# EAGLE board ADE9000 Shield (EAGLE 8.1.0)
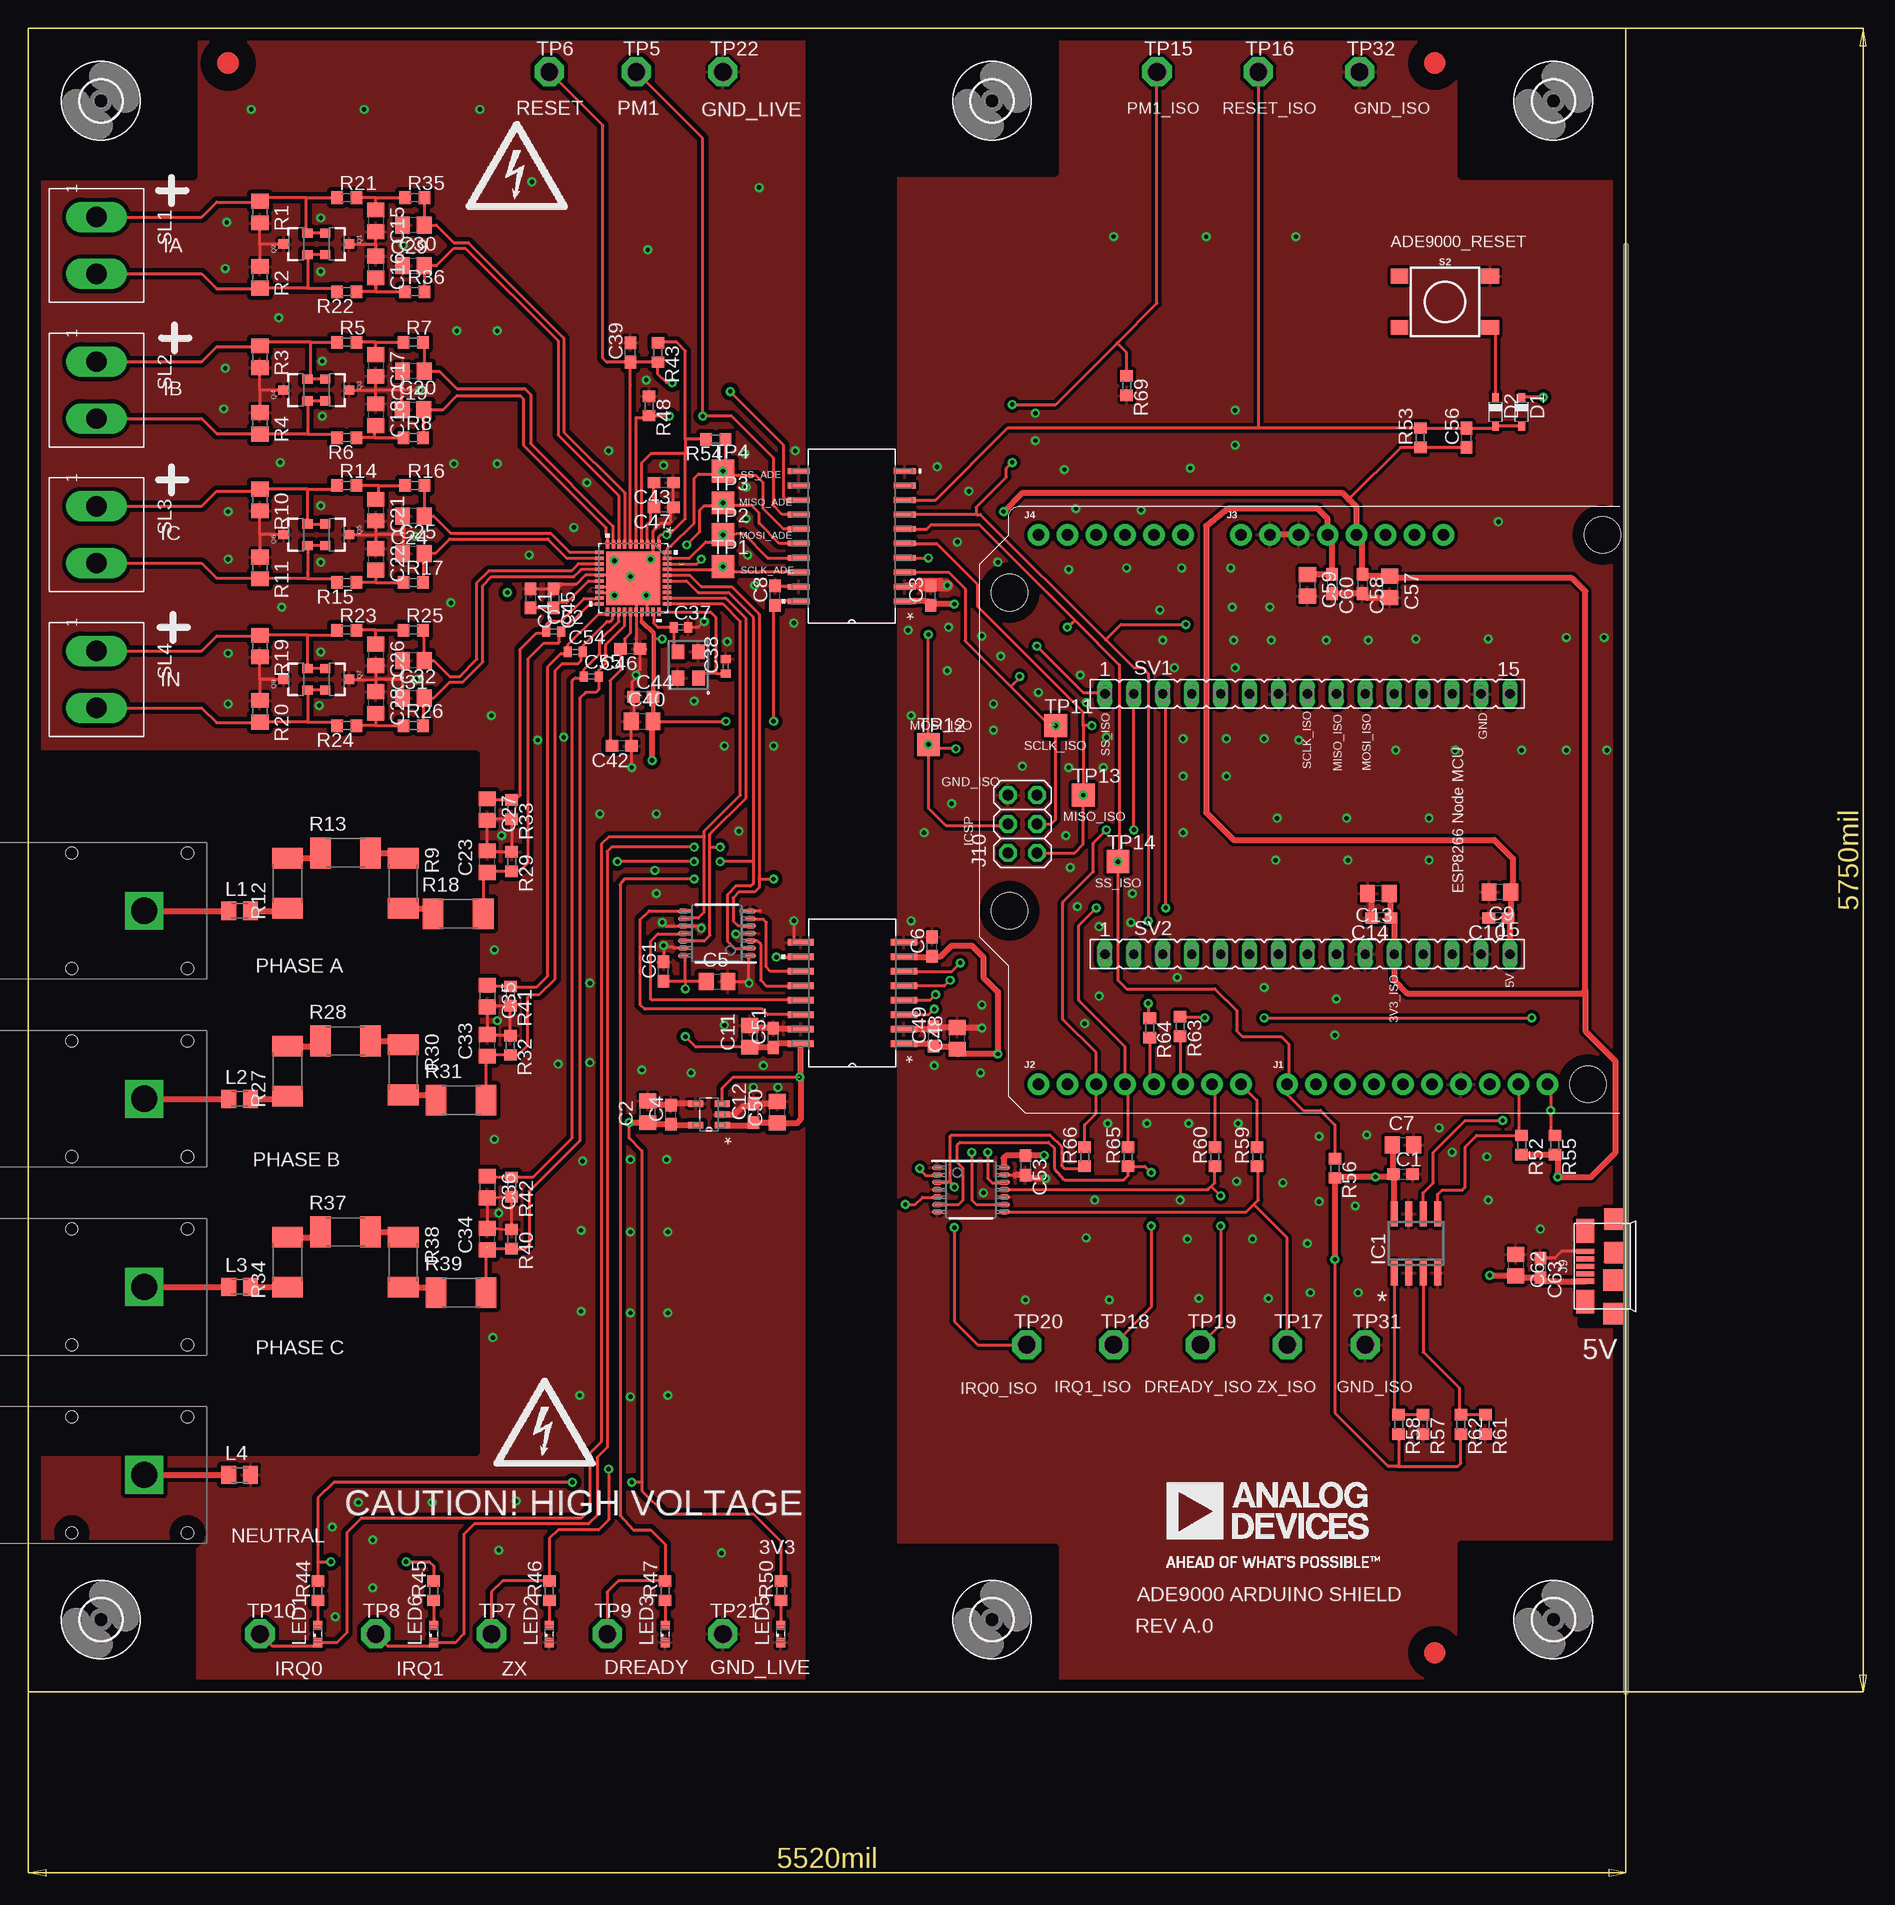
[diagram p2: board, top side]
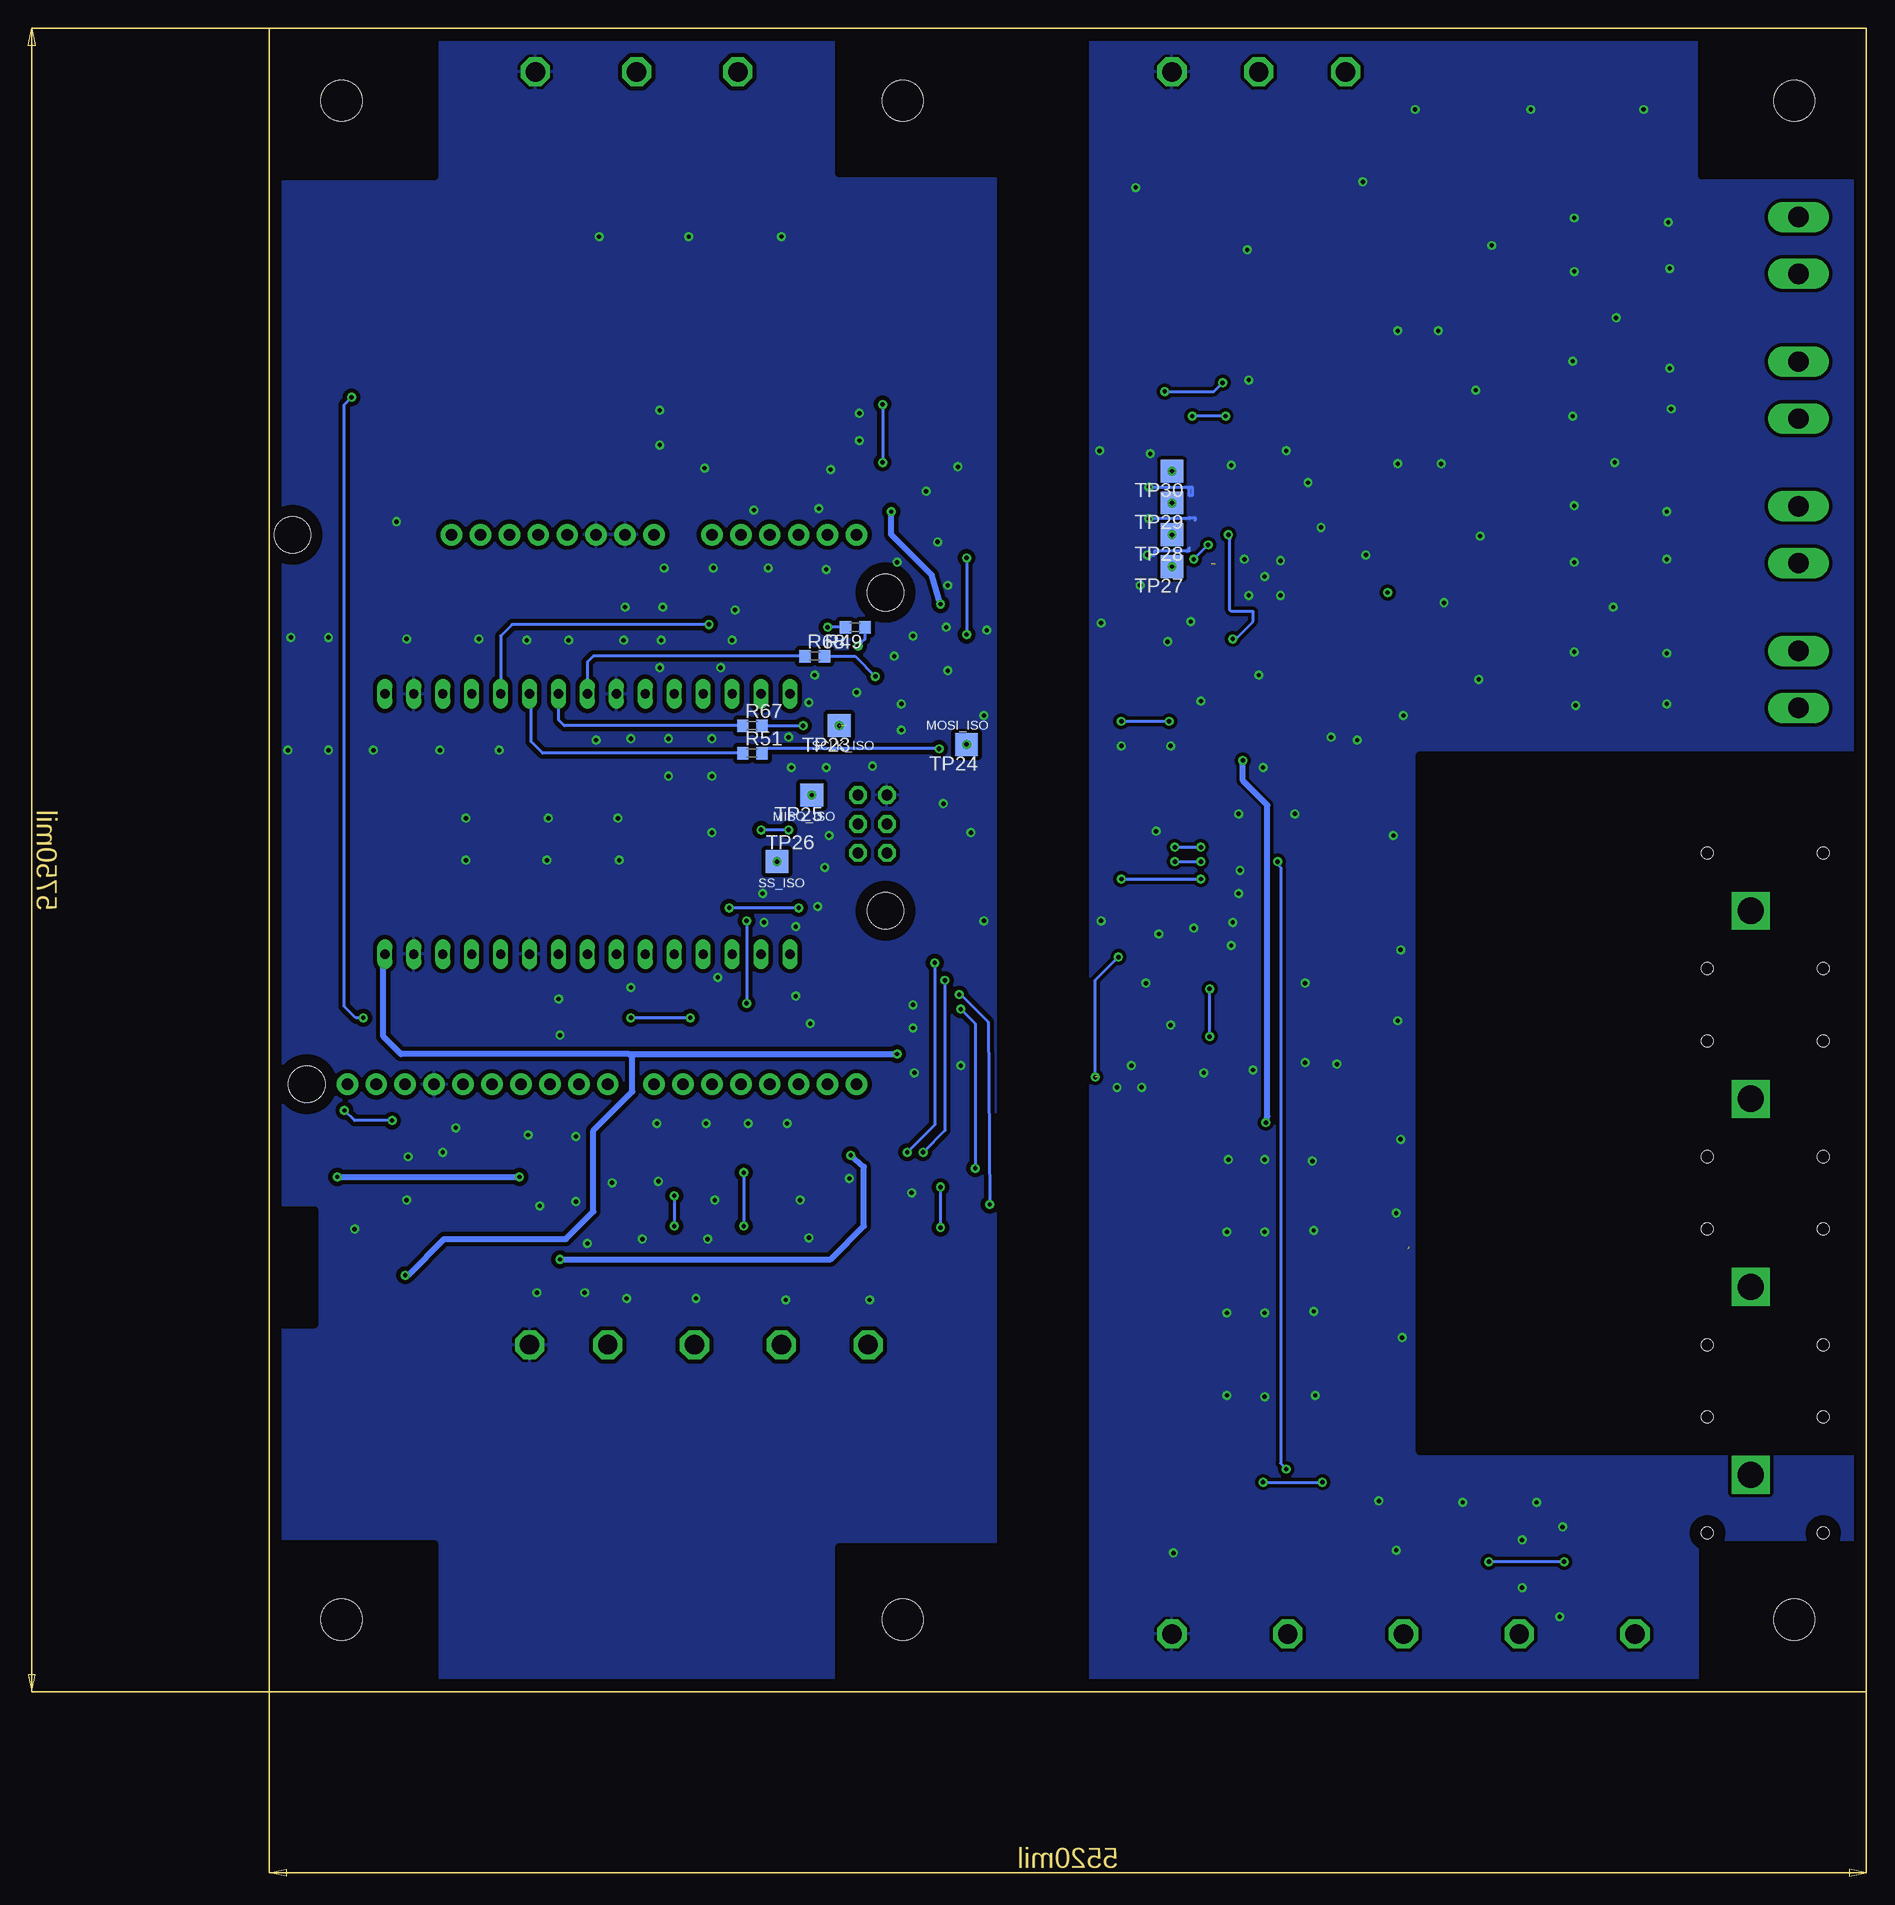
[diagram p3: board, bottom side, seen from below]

Size 161.34 x 162.23 mm. Coordinates in mm from the lower left corner, seen from the top.
Outline: 0,16.18 140.21,16.18 140.21,162.23 0,162.23 0,16.18
Copper layers (1*16): Top 0.035mm / dielectric 1.5mm / Bottom 0.035mm
Design rules "default": minimum track width 10mil, minimum drill 24mil, track to track 8mil, track to pad 8mil, pad to pad 8mil, via to via 8mil, smd to smd 8mil, copper to edge 40mil, drill to drill 8mil, minimum pad ring 10mil, minimum via ring 8mil, stop-mask expansion 4mil, vias tented up to drill 0mil, thermal gap 10mil
Holes 3.2 mm at 136.91,69.52 86.11,84.75 86.11,112.69 138.18,117.77
tRestrict: area 0,37.3 to 39.2,98.5; area 68.6,111.7 to 75.9,125.9; area 68.6,82.3 to 75.9,82.5; area 69,72.6 to 75.7,82.3; area 68.6,16.2 to 75.9,72.6; area 68.6,82.3 to 75.9,162.2; area 0.1,16.4 to 14.4,29.1; area 125.7,16.4 to 140,29.1; area 125.7,149.3 to 140,162; area 0.3,149.3 to 14.5,162; area 136.3,48.4 to 139.3,58.5; area 75.9,16.2 to 90.2,28.9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
bRestrict: area 0,37.3 to 39.2,98.5; area 68.6,16.2 to 75.9,162.2; area 0.1,16.4 to 14.4,29.1; area 125.7,16.4 to 140,29.1; area 125.7,149.3 to 140,162; area 0.3,149.3 to 14.5,162; area 136.3,48.4 to 139.3,58.5; area 75.9,16.2 to 90.2,28.9; area 75.9,149.5 to 90.2,162.2

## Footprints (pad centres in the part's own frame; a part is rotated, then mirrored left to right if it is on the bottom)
C0603 = smd 1.1 x 1: 1 -0.85,0; 2 0.85,0
C0805 = smd 1.3 x 1.5: 1 -0.95,0; 2 0.95,0
C0402 = smd 0.7 x 0.9: 1 -0.65,0; 2 0.65,0
SOD323_ST = smd 0.8 x 0.6: A 1.25,0; C -1.25,0
3,6 = hole 3.6: 0,0
SO-08 = smd 0.6 x 2.2: 1 -1.905,-2.6; 2 -0.635,-2.6; 3 0.635,-2.6; 4 1.905,-2.6; 5 1.905,2.6; 6 0.635,2.6; 7 -0.635,2.6; 8 -1.905,2.6
1X10_NO_SILK = drill 1.016 pad 1.88: 1 0,0; 2 2.54,0; 3 5.08,0; 4 7.62,0; 5 10.16,0; 6 12.7,0; 7 15.24,0; 8 17.78,0; 9 20.32,0; 10 22.86,0
1X08_NO_SILK = drill 1.016 pad 1.88: 1 0,0; 2 2.54,0; 3 5.08,0; 4 7.62,0; 5 10.16,0; 6 12.7,0; 7 15.24,0; 8 17.78,0
1X06_NO_SILK = drill 1.016 pad 1.88: 1 0,0; 2 2.54,0; 3 5.08,0; 4 7.62,0; 5 10.16,0; 6 12.7,0
SLB4-I/90 = drill 2.305 pad 2.794 square: P$1 0,0 | hole 1.054: -3.8,-5.08; -3.8,5.08; 6.36,5.08; 6.36,-5.08
USB-MICRO-10103594 = smd 0.4 x 1.6: D+ 0,0; D- -0.65,0; GND 1.3,0; ID 0.65,0; VBUS -1.3,0 | smd 1.9 x 1.9: SHLD1 -1.2,-2.55; SHLD2 1.2,-2.55; SHLD3 -4.15,-2.55; SHLD4 4.15,-2.55 | smd 2.1 x 1.6: SHLD5 3.1,0; SHLD6 -3.1,0
ARDUINO_2X03 = drill 0.95 pad 1.55 octagon: 1 -2.54,-1.27; 2 -2.54,1.27; 3 0,-1.27; 4 0,1.27; 5 2.54,-1.27; 6 2.54,1.27
M0805 = smd 1.3 x 1.6: 1 -0.95,0; 2 0.95,0
SML0603 = smd 0.8 x 0.8: A 0.75,0; C -0.75,0
SOT23-3 = smd 0.8 x 0.9: 1 -0.95,-1; 2 0.95,-1; 3 0,1.1
SMD_4PIN_3.2X2.1 = smd 1.3 x 1.1: 1 -1.15,-0.9; 2 1.15,-0.9; 3 1.15,0.9; 4 -1.15,0.9
R0805 = smd 1.3 x 1.5: 1 -0.95,0; 2 0.95,0
R0603 = smd 1 x 1.1: 1 -0.85,0; 2 0.85,0
R2010 = smd 1.8 x 2.7: 1 -2.2,0; 2 2.2,0
TACTILE_SWITCH_SMD_6.2MM_TALL = smd 1.55 x 1.3: A1 -3.975,-2.25; A2 3.975,-2.25; B1 -3.975,2.25; B2 3.975,2.25
02P = drill 1.778 long: 1 -2.5,0; 2 2.5,0
FE15 = drill 0.813 long: 1 -17.78,0; 2 -15.24,0; 3 -12.7,0; 4 -10.16,0; 5 -7.62,0; 6 -5.08,0; 7 -2.54,0; 8 0,0; 9 2.54,0; 10 5.08,0; 11 7.62,0; 12 10.16,0; 13 12.7,0; 14 15.24,0; 15 17.78,0
TP20SQ = smd 2 x 2: TP 0,0
P1-17 = drill 1.702 pad 2.54 octagon: TP 0,0
CP_40_7 = smd 0.762 x 0.305: 1 -2.972,2.25; 2 -2.972,1.75; 3 -2.972,1.25; 4 -2.972,0.75; 5 -2.972,0.25; 6 -2.972,-0.25; 7 -2.972,-0.75; 8 -2.972,-1.25; 9 -2.972,-1.75; 10 -2.972,-2.25; 21 2.972,-2.25; 22 2.972,-1.75; 23 2.972,-1.25; 24 2.972,-0.75; 25 2.972,-0.25; 26 2.972,0.25; 27 2.972,0.75; 28 2.972,1.25; 29 2.972,1.75; 30 2.972,2.25 | smd 0.305 x 0.762: 11 -2.25,-2.972; 12 -1.75,-2.972; 13 -1.25,-2.972; 14 -0.75,-2.972; 15 -0.25,-2.972; 16 0.25,-2.972; 17 0.75,-2.972; 18 1.25,-2.972; 19 1.75,-2.972; 20 2.25,-2.972; 31 2.25,2.972; 32 1.75,2.972; 33 1.25,2.972; 34 0.75,2.972; 35 0.25,2.972; 36 -0.25,2.972; 37 -0.75,2.972; 38 -1.25,2.972; 39 -1.75,2.972; 40 -2.25,2.972 | smd 4.699 x 4.699: 41 0,0
RI_16_1 = smd 2.306 x 0.561: 1 -4.527,4.445; 2 -4.527,3.175; 3 -4.527,1.905; 4 -4.527,0.635; 5 -4.527,-0.635; 6 -4.527,-1.905; 7 -4.527,-3.175; 8 -4.527,-4.445; 9 4.527,-4.445; 10 4.527,-3.175; 11 4.527,-1.905; 12 4.527,-0.635; 13 4.527,0.635; 14 4.527,1.905; 15 4.527,3.175; 16 4.527,4.445
PW0014A_N = smd 0.95 x 0.45: 1 -2.95,1.95; 2 -2.95,1.3; 3 -2.95,0.65; 4 -2.95,0; 5 -2.95,-0.65; 6 -2.95,-1.3; 7 -2.95,-1.95; 8 2.95,-1.95; 9 2.95,-1.3; 10 2.95,-0.65; 11 2.95,0; 12 2.95,0.65; 13 2.95,1.3; 14 2.95,1.95
UJ_5 = smd 1.321 x 0.559: 1 -1.168,0.95; 2 -1.168,0; 3 -1.168,-0.95; 4 1.168,-0.95; 5 1.168,0.95
RI_20_1 = smd 1.921 x 0.511: 1 -4.65,5.715; 2 -4.65,4.445; 3 -4.65,3.175; 4 -4.65,1.905; 5 -4.65,0.635; 6 -4.65,-0.635; 7 -4.65,-1.905; 8 -4.65,-3.175; 9 -4.65,-4.445; 10 -4.65,-5.715; 11 4.65,-5.715; 12 4.65,-4.445; 13 4.65,-3.175; 14 4.65,-1.905; 15 4.65,-0.635; 16 4.65,0.635; 17 4.65,1.905; 18 4.65,3.175; 19 4.65,4.445; 20 4.65,5.715

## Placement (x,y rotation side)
C1  0.1u  [C0603]  120.65,61.64 0 top
C2  10u  [C0805]  54.36,67.1 90 top
C3  0.1u  [C0603]  79.2,112.44 90 top
C4  0.1u  [C0603]  56.39,66.85 90 top
C5  4.7u  [C0805]  60.45,78.53 0 top
C6  0.1u  [C0603]  79.32,81.61 90 top
C7  4.7u  [C0805]  120.65,64.18 0 top
C8  0.1u  [C0603]  65.53,112.44 90 top
C9  10u  [C0805]  129.16,86.41 180 top
C10  0.1u  [C0603]  129.03,84.12 180 top
C11  10u  [C0805]  63.3,73.73 90 top
C12  0.1u  [C0603]  63.65,67 90 top
C13  10u  [C0805]  118.49,86.28 180 top
C14  0.1u  [C0603]  118.75,84.12 180 top
C15  DNP  [C0805]  30.48,145.33 270 top
C16  DNP  [C0805]  30.48,141.27 270 top
C17  DNP  [C0805]  30.48,132.63 270 top
C18  DNP  [C0805]  30.48,128.32 270 top
C19  0.022u  [C0805]  33.78,132.13 180 top
C20  0.022u  [C0805]  33.76,128.77 0 top
C21  DNP  [C0805]  30.48,119.93 270 top
C22  DNP  [C0805]  30.48,115.62 270 top
C23  0.022u  [C0805]  40.26,89.07 90 top
C24  0.022u  [C0805]  33.78,119.43 180 top
C25  0.022u  [C0805]  33.78,116.12 0 top
C26  DNP  [C0805]  30.48,107.23 270 top
C27  0.022u  [C0805]  40.26,93.64 270 top
C28  DNP  [C0805]  30.48,103.04 270 top
C29  0.022u  [C0805]  33.78,144.95 180 top
C30  0.022u  [C0805]  33.78,141.4 0 top
C31  0.022u  [C0805]  33.78,106.73 180 top
C32  0.022u  [C0805]  33.78,103.42 0 top
C33  0.022u  [C0805]  40.26,72.94 90 top
C34  0.022u  [C0805]  40.26,55.93 90 top
C35  0.022u  [C0805]  40.26,77.26 270 top
C36  0.022u  [C0805]  40.26,60.5 270 top
C37  18p  [C0402]  57.28,109.65 0 top
C38  18p  [C0402]  61.21,106.22 90 top
C39  1u  [C0603]  52.83,133.78 90 top
C40  4.7u  [C0805]  53.87,101.39 0 top
C41  4.7u  [C0603]  44.07,112.19 270 top
C42  4.7u  [C0603]  52.07,99.23 180 top
C43  4.7u  [C0603]  55.75,122.35 180 top
C44  0.1u  [C0603]  53.98,103.55 0 top
C45  0.1u  [C0603]  46.1,112.19 270 top
C46  0.1u  [C0603]  52.83,107.74 180 top
C47  0.1u  [C0603]  55.75,120.19 180 top
C48  10u  [C0805]  81.53,73.55 90 top
C49  0.1u  [C0603]  79.45,73.71 90 top
C50  10u  [C0805]  65.74,67.08 90 top
C51  0.1u  [C0603]  65.38,73.6 90 top
C52  51p  [C0402]  46.1,109.27 0 top
C53  0.1u  [C0603]  87.5,62.4 270 top
C54  51p  [C0402]  48.01,107.49 0 top
C55  51p  [C0402]  49.4,105.33 0 top
C56  1u  [C0603]  126.24,126.28 90 top
C57  10u  [C0805]  119.51,113.2 270 top
C58  0.1u  [C0603]  117.09,113.46 270 top
C59  10u  [C0805]  112.27,113.33 270 top
C60  0.1u  [C0603]  114.43,113.46 270 top
C61  0.1u  [C0603]  55.75,79.42 90 top
C62  22u  [C0805]  130.56,53.64 270 top
C63  0.1u  [C0603]  132.72,53.39 270 top
D1  BAT54WS  [SOD323_ST]  131.06,128.57 270 top
D2  BAT54WS  [SOD323_ST]  128.78,128.57 270 top
DRILEGEND  [DRILEGEND]  not placed on the board
H1  MOUNT-HOLE3.6  [3,6]  6.35,22.52 0 top
H2  MOUNT-HOLE3.6  [3,6]  6.35,155.88 0 top
H3  MOUNT-HOLE3.6  [3,6]  133.86,155.88 0 top
H4  MOUNT-HOLE3.6  [3,6]  133.86,22.52 0 top
H5  MOUNT-HOLE3.6  [3,6]  84.58,22.52 0 top
H6  MOUNT-HOLE3.6  [3,6]  84.58,155.88 0 top
IC1  24LC32A/SN  [SO-08]  121.79,55.55 0 top
J1  [1X10_NO_SILK]  110.49,69.52 0 top
J2  [1X08_NO_SILK]  88.65,69.52 0 top
J3  [1X08_NO_SILK]  106.43,117.77 0 top
J4  [1X06_NO_SILK]  88.65,117.77 0 top
J5  23.3200-22  [SLB4-I/90]  10.16,84.75 180 top
J6  23.3200-22  [SLB4-I/90]  10.16,68.25 180 top
J7  23.3200-22  [SLB4-I/90]  10.16,51.73 180 top
J8  23.3200-21  [SLB4-I/90]  10.16,35.23 180 top
J9  ZX62-AB-5PA(31)  [USB-MICRO-10103594]  136.65,53.54 90 top
J10  [ARDUINO_2X03]  87.25,92.38 90 top
L1  1500  [M0805]  18.54,84.75 0 top
L2  1500  [M0805]  18.54,68.25 0 top
L3  1500  [M0805]  18.54,51.73 0 top
L4  1500  [M0805]  18.54,35.23 0 top
LED1  APT1608LSECK/J3-PRV  [SML0603]  25.4,21.26 90 top
LED2  APT1608LSECK/J3-PRV  [SML0603]  45.72,21.26 90 top
LED3  APT1608LSECK/J3-PRV  [SML0603]  55.88,21.26 90 top
LED5  APT1608LZGCK  [SML0603]  66.04,21.26 90 top
LED6  APT1608LSECK/J3-PRV  [SML0603]  35.56,21.26 90 top
Q1  MMBD4148SE  [SOT23-3]  27.05,143.3 270 top
Q2  MMBD4148SE  [SOT23-3]  23.5,143.3 90 top
Q3  MMBD4148SE  [SOT23-3]  27.05,130.47 270 top
Q4  MMBD4148SE  [SOT23-3]  23.5,130.47 90 top
Q5  MMBD4148SE  [SOT23-3]  27.05,117.77 270 top
Q6  MMBD4148SE  [SOT23-3]  23.5,117.77 90 top
Q7  MMBD4148SE  [SOT23-3]  27.05,105.08 270 top
Q8  ECS-245.7-12-33Q-JES-TR  [SMD_4PIN_3.2X2.1]  57.91,106.34 90 top
Q9  MMBD4148SE  [SOT23-3]  23.5,105.08 90 top
R1  5.1  [R0805]  20.32,146.1 270 top
R2  5.1  [R0805]  20.32,140.38 270 top
R3  5.1  [R0805]  20.32,133.4 270 top
R4  5.1  [R0805]  20.32,127.55 270 top
R5  0  [R0603]  27.94,134.67 0 top
R6  0  [R0603]  27.94,126.28 180 top
R7  1k  [R0603]  33.78,134.67 0 top
R8  1k  [R0603]  33.78,126.28 0 top
R9  200k  [R2010]  32.89,87.17 270 top
R10  5.1  [R0805]  20.32,120.82 270 top
R11  5.1  [R0805]  20.32,114.85 270 top
R12  200k  [R2010]  22.73,87.17 90 top
R13  200k  [R2010]  27.81,89.83 0 top
R14  0  [R0603]  27.94,122.09 0 top
R15  0  [R0603]  27.94,113.58 180 top
R16  1k  [R0603]  33.91,122.09 0 top
R17  1k  [R0603]  33.78,113.58 0 top
R18  200k  [R2010]  37.72,84.5 0 top
R19  5.1  [R0805]  20.32,108 270 top
R20  5.1  [R0805]  20.32,102.28 270 top
R21  0  [R0603]  27.94,147.37 0 top
R22  0  [R0603]  27.94,139.11 180 top
R23  0  [R0603]  27.94,109.39 0 top
R24  0  [R0603]  27.94,101.01 180 top
R25  1k  [R0603]  33.78,109.39 0 top
R26  1k  [R0603]  33.78,101.01 0 top
R27  200k  [R2010]  22.73,70.66 90 top
R28  200k  [R2010]  27.81,73.33 0 top
R29  1k  [R0603]  42.42,89.07 270 top
R30  200k  [R2010]  32.89,70.78 270 top
R31  200k  [R2010]  37.97,68.12 0 top
R32  1k  [R0603]  42.29,72.94 270 top
R33  1k  [R0603]  42.42,93.64 270 top
R34  200k  [R2010]  22.73,53.89 90 top
R35  1k  [R0603]  33.91,147.37 0 top
R36  1k  [R0603]  33.91,139.11 0 top
R37  200k  [R2010]  27.81,56.56 0 top
R38  200k  [R2010]  32.89,53.89 270 top
R39  200k  [R2010]  37.97,51.23 0 top
R40  1k  [R0603]  42.42,55.93 270 top
R41  1k  [R0603]  42.29,77.26 270 top
R42  1k  [R0603]  42.42,60.5 270 top
R43  10k  [R0603]  55.24,133.78 270 top
R44  3k  [R0603]  25.4,25.07 90 top
R45  3k  [R0603]  35.56,25.07 90 top
R46  3k  [R0603]  45.72,25.07 90 top
R47  3k  [R0603]  55.88,25.07 90 top
R48  10k  [R0603]  54.48,129.08 270 top
R49  DNP  [R0603]  88.77,109.65 180 bottom
R50  3k  [R0603]  66.04,25.07 90 top
R51  DNP  [R0603]  97.79,98.6 0 bottom
R52  10k  [R0603]  131.06,64.18 270 top
R53  10k  [R0603]  122.17,126.28 90 top
R54  10k  [R0603]  60.33,126.16 180 top
R55  10k  [R0603]  133.99,64.18 270 top
R56  10k  [R0603]  114.68,62.15 270 top
R57  0  [R0603]  122.43,39.67 270 top
R58  DNP  [R0603]  120.27,39.67 270 top
R59  0  [R0603]  107.82,63.17 90 top
R60  0  [R0603]  104.14,63.17 90 top
R61  DNP  [R0603]  127.89,39.67 270 top
R62  0  [R0603]  125.73,39.67 270 top
R63  0  [R0603]  101.09,74.59 270 top
R64  0  [R0603]  98.42,74.47 270 top
R65  0  [R0603]  96.52,63.17 90 top
R66  0  [R0603]  92.71,63.17 90 top
R67  DNP  [R0603]  97.79,101.01 0 bottom
R68  DNP  [R0603]  92.33,107.11 0 bottom
R69  10k  [R0603]  96.39,130.86 270 top
S2  PTS645SM43SMTR92  [TACTILE_SWITCH_SMD_6.2MM_TALL]  124.33,138.22 0 top
SL1  25.161.0253.0  [02P]  5.97,143.18 270 top
SL2  25.161.0253.0  [02P]  5.97,130.47 270 top
SL3  25.161.0253.0  [02P]  5.97,117.77 270 top
SL4  25.161.0253.0  [02P]  5.97,105.08 270 top
SV1  DNI  [FE15]  112.27,103.8 0 top
SV2  DNI  [FE15]  112.27,80.94 0 top
TP1  TPTP20SQ  [TP20SQ]  60.96,114.98 0 top
TP2  TPTP20SQ  [TP20SQ]  60.96,117.77 0 top
TP3  TPTP20SQ  [TP20SQ]  60.96,120.57 0 top
TP4  TPTP20SQ  [TP20SQ]  60.96,123.36 0 top
TP5  TPPAD1-17  [P1-17]  53.34,158.42 0 top
TP6  TPPAD1-17  [P1-17]  45.72,158.42 0 top
TP7  TPPAD1-17  [P1-17]  40.64,21.26 0 top
TP8  TPPAD1-17  [P1-17]  30.48,21.26 0 top
TP9  TPPAD1-17  [P1-17]  50.8,21.26 0 top
TP10  TPPAD1-17  [P1-17]  20.32,21.26 0 top
TP11  TPTP20SQ  [TP20SQ]  90.17,101.01 0 top
TP12  TPTP20SQ  [TP20SQ]  78.99,99.36 0 top
TP13  TPTP20SQ  [TP20SQ]  92.58,94.91 0 top
TP14  TPTP20SQ  [TP20SQ]  95.63,89.07 0 top
TP15  TPPAD1-17  [P1-17]  99.06,158.42 0 top
TP16  TPPAD1-17  [P1-17]  107.95,158.42 0 top
TP17  TPPAD1-17  [P1-17]  110.49,46.66 0 top
TP18  TPPAD1-17  [P1-17]  95.25,46.66 0 top
TP19  TPPAD1-17  [P1-17]  102.87,46.66 0 top
TP20  TPPAD1-17  [P1-17]  87.63,46.66 0 top
TP21  TPPAD1-17  [P1-17]  60.96,21.26 0 top
TP22  TPPAD1-17  [P1-17]  60.96,158.42 0 top
TP23  TPTP20SQ  [TP20SQ]  90.17,101.01 180 bottom
TP24  TPTP20SQ  [TP20SQ]  78.99,99.36 180 bottom
TP25  TPTP20SQ  [TP20SQ]  92.58,94.91 180 bottom
TP26  TPTP20SQ  [TP20SQ]  95.63,89.07 0 bottom
TP27  TPTP20SQ  [TP20SQ]  60.96,114.98 180 bottom
TP28  TPTP20SQ  [TP20SQ]  60.96,117.77 180 bottom
TP29  TPTP20SQ  [TP20SQ]  60.96,120.57 180 bottom
TP30  TPTP20SQ  [TP20SQ]  60.96,123.36 180 bottom
TP31  TPPAD1-17  [P1-17]  117.35,46.66 0 top
TP32  TPPAD1-17  [P1-17]  116.84,158.42 0 top
U1  ADE9000ACPZ  [CP_40_7]  53.09,113.97 270 top
U2  ADUM6404ARIZ  [RI_16_1]  72.31,77.54 180 top
U3  SN74LV4T125PWR  [PW0014A_N]  60.43,82.77 180 top
U4  ADP122AUJZ-3.3-R7  [UJ_5]  59.74,66.87 180 top
U5  ADUM4151BRIZ  [RI_20_1]  72.26,117.65 180 top
U6  SN74LV4T125PWR  [PW0014A_N]  82.73,60.27 0 top

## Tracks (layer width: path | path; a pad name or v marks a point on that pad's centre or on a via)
5V_ADE  (via drill 0.38)  (1 unrouted)
  Top 0.254: U4.3 60.91,69.21 61.85,70.15 67.53,70.15 67.79,70.4 | v65.66,80.69 67.76,80.69 U2.10 | C11.1 58.58,72.78 v57.66,73.71 | 57.66,78.53 v57.66,77.9 | 57.66,78.53 57.66,80.64 U3.14 | C61.1 57.62,78.57 57.66,78.53 | C5.1 57.66,78.53
  Top 0.508: C51.1 65.28,72.53 | C51.1 63.32,72.75 C11.1 | U4.1 63.42,65.92 C12.1 65.71,66.15 C50.1 65.78,66.09 67.44,66.09 67.79,66.44 67.79,70.4 U2.16 65.72,73.1 C51.1
  Bottom 0.254: v67.69,70.15 67.69,78.66 v65.66,80.69 | v57.66,73.71 v57.66,77.9
+3V3  (via drill 0.38)
  Top 0.254: 53.85,110.16 U1.27 | R43.1 55.28,134.67 56.9,134.67 57.66,133.9 57.66,126.16 | 57.66,126.16 57.66,124.89 57.56,124.89 | 57.56,124.89 54.61,124.89 53.84,124.11 U1.4 | C40.2 v61.21,101.39 | v65.41,101.39 65.41,111.21 C8.1 65.87,111.93 U5.20 | 53.85,34.59 53.85,63.67 52.72,64.81 v52.72,66.15 | 53.85,34.59 53.85,33.83 55.88,31.8 63.63,31.8 66.04,29.38 R50.2 | 53.85,34.59 v52.96,34.59 | v47.75,34.59 26.8,34.59 25.4,33.19 25.4,27.61 | 25.4,27.61 R44.2 | 25.4,27.61 v26.54,27.61 | v33.15,27.61 35.18,27.61 35.56,27.22 R45.2 | R54.2 57.66,126.16 | v55.63,108.63 54.86,108.63 | U1.1 55.34,117.61 55.5,117.77 v56.01,117.77 56.26,117.77 57.66,119.17 57.66,124.78 57.56,124.89
  Top 0.381: C40.2 C44.2 54.86,105.91 54.86,108.63 54.86,109.14 53.85,110.16 | 56.39,65.92 C4.1
  Top 0.508: U4.5 56.39,65.92 C4.1 54.36,66 C2.1 v52.72,66.15 | v54.74,97.96 54.74,101.31 C40.2
  Bottom 0.254: v61.21,101.39 v65.41,101.39 | v52.96,34.59 v47.75,34.59 | v26.54,27.61 v33.15,27.61 | v55.63,108.63 55.37,108.63 53.85,110.16 53.85,111.04 55.75,111.04 55.88,111.17 55.88,117.39 v56.01,117.77
  Bottom 0.508: v54.74,97.96 54.74,96.19 52.58,94.03 52.58,66.72 52.59,66.71 v52.72,66.15
AVDDOUT
  Top 0.254: U1.25 52.84,109.14 52.32,108.63 52.32,108.08 C46.2 51.98,105.88 51.05,104.95 51.05,99.4 C42.2 51.44,99.07
DREADY_ADE  (via drill 0.38)
  Top 0.254: 63.05,83.42 U3.5 62.29,83.42 61.85,83.87 61.85,85.9 62.36,86.41 63.75,86.41 64.14,86.79 64.14,87.55 | U1.36 58.04,114.22 59.05,113.2 61.72,113.2 64.14,110.79 64.14,87.55 | 64.14,87.55 v65.41,87.55 | v58.42,87.55 52.32,87.55 51.94,87.04 51.94,31.67 53.09,30.4 54.61,30.4 55.88,29.13 R47.2 51.78,25.91 50.8,24.94 TP9.TP
  Bottom 0.254: v65.41,87.55 v58.42,87.55
DREADY_ARD
  Top 0.254: R60.2 104.14,69.26 J2.7
DREADY_ISO  (via drill 0.38)
  Top 0.254: U6.11 103.53,60.27 103.82,60.56 | 103.82,60.56 104.14,60.88 R60.1 | 103.82,60.56 v104.65,59.74 | v104.65,57.07 104.65,48.43 TP19.TP
  Bottom 0.254: v104.65,59.74 v104.65,57.07
DVDDOUT
  Top 0.254: U1.3 54.34,118.64 54.61,118.92 54.61,119.89 C47.2 C43.2
GND  (via drill 0.38)
  Top 0.254: 20.32,143.18 R1.2 | 20.32,143.18 R2.1 | Q2.3 20.45,143.3 20.32,143.18 | 30.48,143.3 C15.2 | 30.48,143.3 C16.1 | Q1.3 30.48,143.3 | C18.1 30.48,130.47 | 30.48,130.47 C17.2 | Q3.3 30.48,130.47 | 20.32,117.77 R10.2 | 20.32,117.77 R11.1 | 20.32,130.47 R3.2 | 20.32,130.47 R4.1 | Q4.3 20.32,130.47 | Q6.3 20.32,117.77 | C21.2 30.48,117.77 | 30.48,117.77 C22.1 | Q5.3 30.48,117.77 | 20.32,105.08 R19.2 | 20.32,105.08 R20.1 | Q9.3 20.32,105.08 | C26.2 30.48,105.08 | 30.48,105.08 C28.1 | Q7.3 30.48,105.08 | 32.93,117.77 30.48,117.77 | U1.41 54.86,115.74 54.86,116 54.74,116 54.84,116.1 U1.2 54.84,118.13 55.5,118.79 56.26,118.79 56.39,118.92 56.39,119.97 C47.1 C43.1 | U1.28 54.34,112.72 U1.41 | U1.41 53.34,113.72 U1.26 53.34,108.09 C46.1 53.72,107.7 53.72,105.96 53.34,105.58 v53.34,105.46 53.34,105.2 52.96,104.82 52.96,103.72 C44.1 53.12,101.59 C40.1 C42.1 52.96,99.19 v52.96,97.33 | U1.18 51.84,112.72 U1.41 | U1.41 52.34,113.22 U1.17 50.1,113.2 | U1.41 52.84,114.22 U1.15 48.89,114.22 48.13,113.46 46.86,113.46 | 46.86,113.46 46.52,113.46 C45.1 | C41.1 C45.1 | 58.55,107.61 58.55,107.86 Q8.2 | C37.2 58.8,109.65 v59.31,110.16 | C33.2 40.13,74.34 40.17,74.3 | C61.2 v55.75,81.71 55.88,81.58 56.52,81.58 56.62,81.47 U3.13 | U3.1 63.25,80.69 v63.25,78.41 63.12,78.53 C5.2 | v67.18,83.87 67.18,81.83 67.63,81.83 U2.9 | U5.19 65.7,113.2 C8.2 | v55.63,83.74 55.94,83.42 U3.10 58.86,83.42 v59.05,83.23 | U3.4 62.15,82.77 v62.1,82.72 | 64.26,84.75 64.23,84.72 U3.7 62.52,84.72 62.48,84.75 | C45.1 46.44,113.04 46.86,113.46 | 32.77,130.47 30.48,130.47 | 32.77,130.47 32.77,130.6 | 32.77,130.47 32.83,130.47 | 32.83,130.47 C19.2 | C20.1 32.77,128.77 32.77,130.47
  Top 0.254: v34.29,130.47 32.83,130.47 | C24.2 32.93,119.43 32.93,117.77 | C25.1 32.93,116.12 32.93,117.77 | 32.83,105.08 30.48,105.08 | 32.83,105.08 C31.2 | C32.1 32.83,105.08 | C33.2 40.26,73.79 R32.1 R41.2 40.26,76.41 C35.2 C33.2 | C23.2 C27.2 40.26,92.8 R33.2 R29.1 40.26,89.92 C23.2 | C34.2 R40.1 R42.2 C36.2 C34.2
  Top 0.508: U2.15 65.42,74.37 C51.2 63.52,74.45 C11.2 63.4,74.33 | U4.4 56.51,67.82 C4.2 54.71,67.7 C2.2 | U4.2 62,66.87 62.74,67.61 63.41,67.61 C12.2 65.56,67.85 C50.2
  Bottom 0.254: v62.99,119.17 59.44,119.17 59.44,119.3 58.93,119.3 58.93,119.05 | v62.99,121.97 59.18,121.97 59.18,121.2 59.44,121.2 59.44,121.97 | v63.12,116 62.48,116 62.48,116.38 59.44,116.38 59.44,116.63
  other vias: 58.17,70.53 51.44,115.49 54.61,115.62 54.23,112.44 51.44,112.44 52.83,114.09 63.75,113.33 62.87,124.89 32.89,143.18 25.65,145.59 25.65,140.89 25.78,133.02 25.78,128.19 33.91,117.65 25.65,115.36 25.65,120.31 17.53,119.81 17.53,115.62 17.27,132.38 17.14,128.82 17.4,145.21 17.27,141.14 17.53,107.36 17.53,102.92 34.04,105.08 25.65,107.49 25.53,102.79 52.83,62.91 52.83,56.56 52.83,49.45 52.83,42.08 42.8,32.94 35.43,32.81 28.96,32.81 26.67,30.65 26.92,22.78 62.36,91.74 54.99,88.31 30.23,29.51 30.23,25.32 60.83,28.37 37.59,135.68 41.15,135.68 37.34,124 41.15,124 37.08,111.81 22.23,111.42 22.1,124.12 21.97,136.83 19.56,155.11 29.46,155.11 39.62,155.11 44.2,148.76 64.14,148.26 54.36,142.79 40.64,101.9 40.89,81.33 40.89,64.69 40.77,47.29 63.63,69.26 65.79,69.26 61.09,74.72 61.09,99.23 65.41,99.23 67.31,125.14 67.18,110.03 50.93,125.14 47.88,118.41 54.23,131.36 61.34,108.38 53.85,70.78 43.94,116 49.02,122.35 41.15,75.1 41.53,91.36 41.27,58.21 56.01,62.91 56.13,56.56 48.64,62.78 48.51,56.69 48.51,49.58 48.39,42.21 56.13,49.45 56.13,42.21 50.16,93.26 55.12,93.26 55.12,86.28 49.28,78.41 44.7,99.74 46.99,99.99 58.42,103.17 55.75,123.87 64.52,71.17 49.28,71.42 46.48,71.29 41.27,28.62
  pour Top (isolate 0.381): 0.13,162.1 68.45,162.1 68.45,16.3 0.13,16.3
  pour Bottom (isolate 0.305): 0.25,16.43 68.33,16.43 68.33,161.97 0.25,161.97
GNDA  (via drill 0.38)
  Top 0.254: 87.34,61.39 C53.2 | 86.61,61.54 85.68,61.54 U6.13 | 80.39,113.58 80.14,113.84 78.23,113.84 78.23,113.67 78.61,113.29 | J9.GND 134.55,54.84 133.99,54.28 132.75,54.28 C63.1
  Top 0.508: 111.63,117.65 J3.3 J3.2 | C60.2 C58.2 117.45,112.25 C57.2 | C3.2 78.61,113.29 78.36,113.29 77,113.29 U5.2 | v89.28,61.26 87.8,61.26 C53.2 86.61,61.55 86.61,61.54 | U2.2 79.26,74.37 C49.2 81.48,74.56 C48.2 83.66,74.5 v83.69,74.47 | C14.2 117.89,85.92 C13.2 | 80.56,113.29 80.39,113.58
  Top 1.016: 78.36,113.29 80.56,113.29 v80.64,113.33
  other vias: 83.69,76.5 88.39,126.03 88.39,128.44 98.17,66.09 101.85,66.09 94.74,66.09 80.77,109.65 79.76,123.74 82.55,121.58 105.92,125.65 105.92,128.7 92.84,56.05 81.03,94.15 78.61,91.61 80.64,105.84 87.5,50.59 94.87,50.59 102.74,50.72 108.84,50.72 83.82,59.99 77.47,83.87 79.5,71.17 106.17,66.09 93.6,59.36 83.57,70.53 77.22,109.39 77.47,101.9 90.93,123.49 101.98,123.62 111.25,143.94 95.25,143.94 103.38,143.94 81.53,117.14 85.09,115.36 91.44,88.56 101.09,59.36 106.05,61.01 110.11,60.88 83.69,108.88 91.31,114.73 96.39,114.85 101.22,114.85 105.54,114.85 105.66,111.42 105.79,108.5 99.57,108.5 99.31,111.17 85.34,107.11 88.65,103.93 84.71,102.92 84.71,100.63 91.31,97.33 94.36,97.33 101.35,99.87 105.16,99.87 108.46,99.87 111.51,99.74 109.09,108.5 113.92,108.5 117.6,108.5 121.79,108.63 128.14,108.63 138.3,108.76 135,108.76 120.02,98.85 125.22,98.85 131.06,98.85 138.56,98.85 135,98.85 105.92,106.09 100.58,106.09 101.35,96.57 105.16,96.57 101.35,91.61 96.9,86.28 92.08,85.14 92.71,74.85 91.06,91.36 94.61,99.99 87.25,97.45 96.77,83.74 93.98,83.36 93.98,77.26 100.84,78.91 108.46,78.02 124.97,63.55 123.83,65.7 117.47,65.07 113.28,64.94 113.28,59.23 116.46,58.85 112.27,55.55 112.52,51.23 116.71,51.23 132.72,56.81 97.66,119.93 91.95,120.06 129.03,118.92 128.02,63.17 128.14,59.36 109.6,92.88 115.7,92.88 109.47,89.2 115.82,89.2 122.94,92.88 122.94,89.2 114.81,77.01 114.68,73.83 92.33,105.46 108.97,111.42 92.84,103.04 101.73,55.93 107.44,55.93
  pour Top (isolate 0.305): 76.07,16.3 140.08,16.3 140.08,162.1 76.07,162.1
  pour Bottom (isolate 0.381): 76.2,16.43 76.2,161.97 140.08,161.97 140.08,16.43
IAN
  Top 0.254: U1.8 51.82,116.96 51.82,121.2 46.48,126.54 46.48,134.79 38.35,142.92 37.34,142.92 35.81,141.4 C30.2 34.76,141.4 R36.2
IAP
  Top 0.254: U1.7 52.32,116.95 52.32,121.46 46.99,126.79 46.99,135.05 38.61,143.43 37.34,143.43 35.81,144.95 C29.1 34.73,147.37 R35.2
IBN
  Top 0.254: U1.10 50.83,116.95 50.83,117.65 50.67,117.8 50.67,118.41 43.43,125.65 43.43,129.71 43.18,129.97 37.59,129.97 36.4,128.77 C20.2 34.71,126.28 R8.2 34.61,126.69
IBP
  Top 0.254: U1.9 51.31,116.97 51.31,118.54 44.07,125.78 44.07,130.09 43.56,130.6 37.59,130.6 36.07,132.13 C19.1 34.73,134.67 R7.2
ICN
  Top 0.254: U1.12 50.09,115.74 47.24,115.74 45.59,117.39 36.96,117.39 35.69,116.12 C25.2 34.63,116.12 R17.2
ICP
  Top 0.254: U1.11 50.08,116.25 47.5,116.25 45.85,117.9 37.08,117.9 35.56,119.43 C24.1 34.73,122.09 R16.2
INN
  Top 0.254: R26.2 C32.2 35.56,103.42 36.96,104.82 38.1,104.82 39.88,106.6 39.88,113.33 40.64,114.09 47.88,114.09 48.5,114.72 U1.14
INP
  Top 0.254: R25.2 C31.1 35.56,106.73 36.96,105.33 37.85,105.33 39.37,106.85 39.37,113.58 40.39,114.6 47.62,114.6 48.24,115.22 U1.13
IRQ0_ADE
  Top 0.254: U1.31 60.92,111.72 62.48,110.16 62.48,94.91 59.31,91.74 59.31,91.23 | U3.9 58.28,84.12 58.8,84.12 59.31,84.63 59.31,91.23 | 59.31,91.23 50.93,91.23 50.29,90.6 50.29,38.15 49.28,37.13 49.28,32.18 48.51,31.41 29.21,31.41 27.94,30.15 27.94,21.38 27.05,20.49 25.41,20.49 LED1.C 25.13,20.24 21.34,20.24 TP10.TP
IRQ0_ARD  (via drill 0.38)
  Top 0.254: R66.2 92.71,65.96 93.73,66.97 J2.3 93.73,72.31 90.81,75.23 90.81,85.52 93.47,88.18 93.47,90.72 v94.61,91.87 | v97.03,91.87 SV1.2
  Bottom 0.254: v94.61,91.87 v97.03,91.87
IRQ0_ISO  (via drill 0.38)
  Top 0.254: U6.3 80.69,60.92 80.9,61.13 | 80.9,61.13 80.9,64.94 81.03,65.07 89.66,65.07 90.68,64.05 90.68,62.4 90.93,62.15 92.54,62.15 | R66.1 92.42,62.02 | 92.54,62.15 R66.1 | 92.54,62.15 R66.1 | 80.9,61.13 80.9,60.88 v81.28,60.5 | v81.28,56.94 81.28,48.69 83.31,46.66 TP20.TP
  Bottom 0.254: v81.28,60.5 v81.28,56.94
IRQ1_ADE  (via drill 0.38)
  Top 0.254: U1.32 61.19,112.22 62.99,110.41 62.99,94.66 59.82,91.49 59.82,90.34 | U3.12 58.27,82.09 59.31,82.09 59.82,82.6 59.82,90.34 | 59.82,90.34 v60.71,90.34 | v58.42,90.34 51.18,90.34 50.8,89.96 50.8,37.64 49.91,36.75 49.91,31.67 49.15,30.91 39.12,30.91 38.23,30.02 38.23,21.26 37.47,20.49 35.57,20.49 LED6.C 35.29,20.24 31.5,20.24 TP8.TP
  Bottom 0.254: v60.71,90.34 v58.42,90.34
IRQ1_ARD  (via drill 0.38)
  Top 0.254: R65.2 96.52,69.26 J2.4 96.27,72.06 | 96.27,72.06 96.27,72.18 | v99.82,85.01 99.82,103.55 SV1.3 | 96.27,72.06 96.27,72.82 92.2,76.88 92.2,83.48 v93.73,85.01
  Bottom 0.254: v93.73,85.01 v99.82,85.01
IRQ1_ISO  (via drill 0.38)
  Top 0.254: U6.6 80.9,58.97 | 80.9,58.97 81.15,58.97 | v98.55,61.77 98,62.31 R65.1 96.52,61.51 96.14,61.13 90.93,61.13 90.04,62.15 90.04,63.93 89.53,64.44 81.79,64.44 81.53,64.18 81.53,62.66 82.04,62.15 82.04,59.36 81.66,58.97 80.9,58.97 | v98.55,57.07 98.55,49.96 TP18.TP
  Bottom 0.254: v98.55,61.77 v98.55,57.07
MISO_ADE  (via drill 0.38)  (1 unrouted)
  Top 0.254: U1.38 57.51,115.22 | U5.16 65.91,117.01 64.14,118.79 64.14,119.68 63.5,120.31 61.21,120.31 TP29.TP 60.71,120.31 59.31,120.31 58.93,119.93 58.93,118.03 v57.78,116.89 | 57.15,115.22 58.65,115.22 v59.05,115.62
  Bottom 0.254: v59.05,115.62 v57.78,116.89
  other vias: 60.96,120.57
MISO_ISO  (via drill 0.38)
  Top 0.254: U5.5 79.7,117.01 83.31,113.41 83.31,111.48 92.58,102.2 92.58,101.01 | J10.1 91.82,89.83 92.58,90.6 TP25.TP 92.58,101.01 | v93.34,101.01 92.58,101.01
  Bottom 0.254: R67.2 v93.34,101.01
  other vias: 92.58,94.91
MOSI_ADE  (via drill 0.38)
  Top 0.254: TP28.TP 60.83,117.77 | TP28.TP 62.74,117.9 64.9,115.74 U5.17 | TP28.TP 60.2,117.14 59.44,117.14 58.01,115.72 U1.39
  other vias: 60.96,117.77
MOSI_ISO  (via drill 0.38)
  Top 0.254: U5.4 v78.99,115.74 | J10.4 85.85,92.25 80.52,92.25 78.99,93.77 TP24.TP | TP24.TP v78.99,109.01 | 79.76,99.49 79.63,99.36 TP24.TP | v81.41,98.98 79.38,98.98 TP24.TP
  Bottom 0.254: v78.99,115.74 v78.99,109.01 | v81.41,98.98 96.69,98.98 R51.2
  other vias: 78.99,99.36
N$1
  Top 0.254: U1.29 54.86,110.97 54.86,110.03 55.24,109.65 C37.1 56.63,107.88 Q8.3
N$2
  Top 0.254: U1.30 59.87,110.99 60.33,110.54 60.33,105.69 60.45,105.57 | 60.45,105.57 C38.1 | 60.45,105.57 59.19,105.57 Q8.1
N$3
  Top 0.254: SL2.1 15.2,132.97 16.51,134.28 20,134.28 R3.1 20.32,134.67 24.77,134.67 | 24.77,134.67 R5.1 | 24.77,134.67 24.77,131.43 Q4.2 Q3.1
N$4
  Top 0.254: SL2.2 15.2,127.97 16.51,126.66 20,126.66 R4.2 24.51,126.6 | Q3.2 Q4.1 24.51,127.17 | 24.51,127.17 24.51,126.98 | 24.51,126.6 27.09,126.6 R6.2 | 24.51,127.17 24.51,126.6
N$6
  Top 0.254: 30.35,126.28 R6.1 | 30.35,126.28 R8.1 | C18.2 30.35,127.37 30.35,126.28
N$7
  Top 0.254: SL1.1 15.2,145.68 16.51,146.99 20,146.99 R1.1 20.32,147.37 24.38,147.37 | Q1.1 Q2.2 24.38,144.25 24.38,147.37 | 24.38,147.37 R21.1
N$8
  Top 0.254: R61.1 R62.1 125.6,40.65 125.6,42.84 122.43,46.02 IC1.3
N$9
  Top 0.254: 30.48,134.67 R5.2 | 30.48,134.67 R7.1 | C17.1 30.48,134.67
N$11
  Top 0.254: SL3.1 15.2,120.27 16.51,121.58 20,121.58 R10.1 24.51,121.77 | 24.13,118.72 Q6.2 | Q6.2 Q5.1 | Q6.2 24.51,121.77 | 24.51,121.77 27.09,121.77 R14.1
N$13
  Top 0.254: SL3.2 15.2,115.27 16.51,113.97 20,113.97 R11.2 24.51,113.9 | Q5.2 Q6.1 24.51,114.47 | 24.51,114.47 24.51,114.28 | 24.51,113.9 27.09,113.9 R15.2 | 24.51,114.47 24.51,113.9
N$14
  Top 0.254: 30.48,139.37 C16.2 30.48,139.11 | 30.48,139.11 R22.1 | 30.48,139.11 R36.1
N$15
  Top 0.508: J8.P$1 L4.1
N$16
  Top 0.254: R63.2 101.09,69.77 J2.6
N$17
  Top 0.254: 30.48,113.58 R15.1 | 30.48,113.58 R17.1 | C22.2 30.48,113.58
N$18
  Top 0.254: 30.73,122.09 R14.2 | 30.73,122.09 R16.1 | C21.1 30.73,120.88 30.73,122.09
N$19
  Top 0.254: R46.1 LED2.A
N$21
  Top 0.254: SL4.1 15.2,107.58 16.51,108.88 20,108.88 R19.1 24.51,108.95 | Q7.1 Q9.2 24.51,108.95 | 24.51,108.95 27.09,108.95 R23.1
N$22
  Top 0.254: SL4.2 15.2,102.58 16.51,101.27 20,101.27 R20.2 24.51,101.33 | Q7.2 Q9.1 24.51,101.33 | 24.51,101.33 27.09,101.33 R24.2
N$23  (via drill 0.38)
  Top 0.254: v88.52,108 92.58,103.93 94.36,103.93 SV1.1
  Bottom 0.254: R49.1 87.92,108.59 v88.52,108
N$24
  Top 0.254: 30.48,101.01 R24.1 | 30.48,101.01 R26.1 | C28.2 30.48,101.01
N$25
  Top 0.254: 30.48,109.39 R23.2 | 30.48,109.39 R25.1 | C26.1 30.48,109.39
N$27
  Top 0.254: R44.1 LED1.A
N$28
  Top 0.254: R45.1 LED6.A
N$29
  Top 0.254: R47.1 LED3.A
N$30
  Top 0.254: U2.14 64.87,75.64 64.39,76.12 54.1,76.12 53.72,76.5 53.72,83.99 54.48,84.75 58.21,84.75 U3.8
N$31
  Top 0.254: U2.13 54.71,76.91 54.61,77.01 54.61,82.09 55.24,82.72 58.19,82.72 U3.11
N$32
  Top 0.254: 22.52,68.25 R27.1
  Top 0.508: L2.2 22.52,68.25
N$33
  Top 0.254: 25.15,72.86 R28.1
  Top 0.508: R27.2 25.15,72.86
N$34
  Top 0.254: 32.55,73.33 R30.1
  Top 0.508: R28.2 32.55,73.33
N$35
  Top 0.254: 22.52,84.75 R12.1
  Top 0.508: L1.2 22.52,84.75
N$36
  Top 0.254: 25.15,89.37 R13.1
  Top 0.508: R12.2 25.15,89.37
N$37
  Top 0.254: 32.43,89.83 R9.1
  Top 0.508: R13.2 32.43,89.83
N$38
  Top 0.254: 35.6,84.97 R18.1
  Top 0.508: R9.2 35.6,84.97
N$39
  Top 0.254: D2.C 128.78,135.5 S2.A2
N$40
  Top 0.254: SL1.2 15.2,140.68 16.51,139.37 20,139.37 R2.2 24.51,139.43 | Q1.2 Q2.1 24.51,139.43 | 24.51,139.43 27.09,139.43 R22.2
N$41
  Top 0.254: 30.48,146.99 C15.1 30.48,147.37 | 30.48,147.37 R21.2 | 30.48,147.37 R35.1
N$42
  Top 0.254: 35.6,68.58 R31.1
  Top 0.508: R30.2 35.6,68.58
N$43  (via drill 0.38)
  other vias: 42.04,112.69
N$44
  Top 0.254: U3.3 63.97,82.12 64.26,81.83 64.26,78.66 64.77,78.15 67.06,78.15 67.18,78.28 67.69,78.28 U2.12
N$45
  Top 0.254: 22.69,51.73 R34.1
  Top 0.508: L3.2 22.69,51.73
N$46
  Top 0.254: 25.15,56.09 R37.1
  Top 0.508: R34.2 25.15,56.09
N$47
  Top 0.254: 32.43,56.56 R38.1
  Top 0.508: R37.2 32.43,56.56
N$48
  Top 0.254: 35.6,51.69 R39.1
  Top 0.508: R38.2 35.6,51.69
N$49
  Top 0.254: U2.11 65.13,79.45 64.77,79.8 64.77,83.74 64.52,83.99 63.46,83.99 U3.6
N$50
  Top 0.254: R50.1 LED5.A
N$52
  Bottom 0.254: SV1.8 112.27,106.6 111.76,107.11 R68.1
N$53
  Bottom 0.254: R67.1 114.3,101.01 114.81,101.52 SV1.9
N$55
  Bottom 0.254: R51.1 116.2,98.6 117.22,99.61 117.22,103.68 SV1.10
N$57  (via drill 0.38)
  Top 0.254: U2.3 79.02,75.64 v79.5,76.12 | 79.71,61.64 U6.2 79.72,61.51 78.74,61.51 78.23,62.02 v78.23,62.15
  Bottom 0.254: v79.5,76.12 78.23,74.85 v78.23,62.15
N$58  (via drill 0.38)
  Top 0.254: U2.4 79.15,76.91 v79.63,77.39 | 79.66,59.74 U6.5 79.77,59.61 78.49,59.61 77.85,58.97 v76.96,58.97
  Bottom 0.254: v79.63,77.39 79.5,77.39 77.09,74.98 v76.96,58.97
N$59  (via drill 0.38)
  Top 0.254: U2.5 80.42,78.18 v80.9,78.66 | v82.8,63.55 82.8,59.36 83.19,58.97 U6.9
  Bottom 0.254: v80.9,78.66 80.9,65.45 v82.8,63.55
N$60  (via drill 0.38)
  Top 0.254: U2.6 81.05,79.45 v81.79,80.18 | v84.2,63.55 84.2,61.26 84.58,60.88 85.64,60.88 U6.12
  Bottom 0.254: v81.79,80.18 81.79,65.96 v84.2,63.55
N$67
  Top 0.508: J5.P$1 L1.1
N$68
  Top 0.508: J6.P$1 L2.1
N$69
  Top 0.508: J7.P$1 L3.1
N$76
  Top 0.254: IC1.1 119.89,40.9 R58.1 R57.1
PM1_ADE  (via drill 0.38)
  Top 0.254: U1.5 53.34,128.06 54.32,128.06 R48.2 56.22,128.23 v56.26,128.19 | U5.14 66.17,119.55 65.41,120.31 65.41,124.51 61.72,128.19 v59.18,128.19 59.18,152.57 TP5.TP
  Bottom 0.254: v56.26,128.19 v59.18,128.19
PM1_ARD
  Top 0.254: R64.2 98.42,69.9 J2.5
PM1_ISO  (via drill 0.38)
  Top 0.254: v86.36,129.21 90.17,129.21 95.57,134.6 | 95.57,134.6 99.06,138.09 TP15.TP | 83.19,119.55 U5.7 | 83.19,119.55 83.57,119.55 94.55,108.57 | 83.19,119.55 83.19,120.19 85.85,122.85 85.85,123.61 v86.36,124.12 | 95.57,134.6 96.39,133.78 R69.1 | 94.55,108.57 95.89,109.9 v101.6,109.9 | 94.55,108.57 97.03,106.09 97.79,106.09 98.3,105.58 v98.3,83.87 | v98.3,76.63 98.3,75.45 R64.1
  Bottom 0.254: v86.36,129.21 v86.36,124.12 | SV1.11 119.89,108.88 118.87,109.9 v101.6,109.9 | v98.3,83.87 v98.3,76.63
REF
  Top 0.254: U1.16 49.15,113.71 47.24,111.81 46.57,111.81 C45.2 C41.2
RESET_ADE  (via drill 0.38)
  Top 0.254: U1.6 52.84,130.87 C39.1 | C39.1 R43.2 55.24,131.87 56.01,131.11 v56.52,131.11 | C39.1 50.76,132.93 50.42,133.27 50.42,153.72 TP6.TP | U5.13 66.55,120.82 66.29,121.08 66.29,125.65 v61.59,130.35
  Bottom 0.254: v61.59,130.35 57.28,130.35 v56.52,131.11
RESET_ARD  (via drill 0.38)
  Top 0.254: R63.1 103.54,75.45 v103.25,75.36 | v108.46,75.36 v131.95,75.36 | v132.97,129.84 131.08,129.84 D1.C
  Bottom 0.254: v103.25,75.36 v108.46,75.36 | v131.95,75.36 132.59,75.36 133.6,76.37 133.6,129.21 v132.97,129.84
RESET_ISO
  Top 0.254: U5.8 79.63,120.82 85.98,127.17 107.95,127.17 | TP16.TP 107.95,127.17 | 107.95,127.17 122.14,127.17 R53.2 C56.2 128.59,127.13 D2.A D1.A
SCL_ARDUINO  (via drill 0.38)
  Top 0.254: IC1.6 122.43,59.99 123.32,60.88 123.32,63.55 126.11,66.34 v129.41,66.34 | v133.6,67.23 133.6,69.26 J1.10 | v133.6,67.23 133.6,66.72 | 134.37,65.16 R55.1 133.6,65.41 v133.6,67.23
  Bottom 0.254: v133.6,67.23 132.72,66.34 v129.41,66.34
SCLK_ADE  (via drill 0.38)
  Top 0.254: U1.37 60.44,114.72 60.64,114.92 | 60.64,114.92 TP27.TP | U5.18 61.09,114.47 60.64,114.92
  other vias: 60.96,114.98
SCLK_ISO  (via drill 0.38)  (1 unrouted)
  Top 0.254: U5.3 80.8,114.47 82.22,113.05 82.22,108.45 86.23,104.44 | 86.23,104.44 89.61,101.06 | v87,105.33 87,105.2 86.23,104.44 | J10.3 89.79,92.38 90.17,92.76 TP23.TP
  Bottom 0.254: v87,105.33 88.77,107.11 R68.2
  other vias: 90.17,101.01
SDA_ARDUINO
  Top 0.254: J1.9 130.81,65.28 R52.1 127.13,65.03 126.11,64.02 126.11,60.5 125.86,60.24 124.08,60.24 123.7,59.86 IC1.5 123.83,58.27
SS_ADE  (via drill 0.38)
  Top 0.254: TP30.TP 60.83,123.11 58.8,123.11 58.42,122.73 58.42,118.79 56.39,116.76 56.26,116.76 56.06,116.56 U1.40 | U5.15 66.29,118.28 64.52,120.06 64.52,122.35 63.88,122.98 61.21,122.98 TP30.TP | R54.1 61.17,123.45 TP30.TP
  other vias: 60.96,123.36
SS_ISO  (via drill 0.38)
  Top 0.254: 110.62,69.39 J1.1 110.49,69.01 | 95.76,89.2 TP26.TP | TP26.TP 96.01,89.45 95.76,89.71 95.76,106.34 91.89,110.22 | 91.89,110.22 83.44,118.66 79.25,118.66 78.87,118.28 U5.6 | 110.49,69.01 110.49,68.63 111.89,67.23 113.41,67.23 114.68,65.96 R56.1 | v91.19,109.65 91.89,110.22 | TP26.TP 95.63,78.66 96.39,77.9 104.14,77.9 106.05,75.99 106.05,74.21 106.55,73.71 109.98,73.71 110.62,73.07 110.62,69.13 110.49,69.01
  Bottom 0.254: R49.2 v91.19,109.65
  other vias: 95.63,89.07
V+  (via drill 0.38)
  Top 0.254: 87.42,63.17 C53.1 | C56.1 R53.1 120.44,125.43 115.89,120.89 | v114.68,54.15 114.68,40.69 119.38,35.99 120.14,35.99 | 120.14,35.99 125.48,35.99 125.73,36.24 R62.2 | R58.2 120.27,36.11 120.14,35.99
  Top 0.508: 79.49,111.55 C3.1 79.11,111.93 78.74,111.93 | 78.74,111.93 U5.1 | v81.28,111.68 78.99,111.68 78.74,111.93 | v89.15,63.29 87.54,63.29 C53.1 85.81,63.25 85.6,63.04 85.6,62.3 U6.14 | v85.6,119.81 87.25,121.46 115.32,121.46 115.89,120.89 116.59,120.19 J3.5 117.09,117.27 C58.1 117.25,114.15 C57.1 119.69,113.97 135.51,113.97 136.65,112.82 136.65,77.77 | C14.1 119.89,84.08 | 119.72,86.43 C13.1 119.59,86.12 C14.1 | C14.1 119.89,83.83 SV2.11 119.89,78.66 121.03,77.52 136.4,77.52 136.65,77.77 | C1.1 119.55,61.39 v118.24,61.39 114.77,61.39 R56.2 v114.68,54.15 | IC1.8 119.89,61.55 C1.1 | C1.1 119.8,64.08 C7.1 | R52.2 R55.2 134.24,63.08 v134.24,61.39 137.16,61.39 139.32,63.55 139.32,71.55 136.65,74.21 136.65,77.77
  Bottom 0.508: v89.15,63.29 88.01,62.28 88.01,57.07 90.93,54.15 v114.68,54.15 | v81.28,111.68 82.04,114.22 85.62,117.8 85.62,119.78 v85.6,119.81 | v134.24,61.39 v118.24,61.39
VAN
  Top 0.254: 42.29,94.66 42.04,94.41 42,94.41 R33.1 | R33.1 42.76,94.49 43.18,94.91 43.18,107.74 44.58,109.14 45.32,109.14 C52.1 45.47,109.28 45.47,109.9 45.72,110.16 46.74,110.16 48.77,112.19 50.09,112.19 U1.19 | R33.1 40.26,94.49 C27.1
VAP
  Top 0.254: U1.20 50.08,111.68 49.28,111.68 48.01,110.41 47.88,110.41 47.39,109.92 C52.2 | 39.88,85.43 R18.2 39.92,88.12 C23.1 40.26,88.22 R29.2 42,88.31 43.18,88.31 43.81,88.95 43.81,106.85 45.21,108.25 46.48,108.25 46.61,108.38 46.61,109.12 C52.2 | 46.86,109.15 C52.2
VBN
  Top 0.254: 50.78,111.04 U1.21 50.63,110.79 50.04,110.79 47.36,108.11 C54.1 47.23,107.36 46.74,107.36 45.59,106.22 45.59,79.04 44.58,78.02 42.38,78.02 R41.1 40.26,78.11 C35.1
VBP
  Top 0.254: R31.2 40.17,72.43 C33.1 40.26,72.09 R32.2 42.97,72.09 43.81,72.94 43.81,77.14 44.07,77.39 44.83,77.39 46.23,78.79 46.23,105.84 46.86,106.47 48.26,106.47 48.51,106.73 48.51,107.35 C54.2 48.66,108.01 50.8,110.16 51.05,110.16 51.31,110.41 51.31,110.97 U1.22
VCC  (via drill 0.38)
  Top 0.254: 134.11,52.24 134.14,52.21
  Top 0.508: C59.1 112.3,114.31 C60.1 114.43,117.39 J3.4 114.05,119.17 113.16,120.06 105.28,120.06 103.38,118.54 103.38,93.39 105.79,90.98 128.65,90.98 130.3,89.33 130.3,87.04 130.18,86.91 130.18,86.47 C9.1 130.11,84.35 C10.1 130.05,83.95 SV2.15 | U2.1 79.21,73.1 C49.1 81.28,72.86 C48.1 81.58,72.18 v85.09,72.18 85.09,77.64 83.82,78.91 83.82,80.69 82.8,81.71 81.03,81.71 80.07,80.75 C6.1 79.32,80.72 U2.7 | J9.VBUS 136.63,52.21 134.14,52.21 132.72,52.21 C63.2 130.71,52.54 C62.2 128.33,52.69 v128.27,52.75
  Bottom 0.508: SV2.15 130.18,80.82 130.18,73.71 128.65,72.18 108.58,72.18 | 108.58,72.18 v85.09,72.18 | 108.58,72.18 108.33,71.93 108.33,68.88 111.76,65.45 111.76,58.34 114.17,55.93 124.84,55.93 128.02,52.75 v128.27,52.75
VCN
  Top 0.254: U1.23 51.82,110.97 51.82,110.16 50.16,108.5 50.16,107.36 48.75,105.95 C55.1 48.63,105.2 48.01,105.2 47.75,104.95 47.75,64.82 44.28,61.35 R42.1 40.26,61.35 C36.1
VCP  (1 unrouted)
  Top 0.254: 52.32,110.98 U1.24 52.34,109.79 50.67,108.12 50.67,106.47 50.05,105.85 C55.2 50.04,105.31 50.04,104.19 49.78,103.93 48.9,103.93 48.39,103.42 48.39,64.56 43.94,60.12 43.94,55.42 43.56,55.04 42.46,55.04 R40.2 40.26,55.08 C34.1 | R39.2 40.17,55.24
ZX_ADE  (via drill 0.38)
  Top 0.254: U1.35 57.78,113.72 58.8,112.69 61.47,112.69 63.63,110.54 63.63,89.07 | U3.2 62.84,81.47 62.82,81.45 61.98,81.45 61.34,82.09 61.34,86.15 62.1,86.91 63.37,86.91 63.63,87.17 63.63,89.07 | 63.63,89.07 v60.71,89.07 | TP7.TP 40.64,24.94 41.62,25.91 R46.2 45.72,29.64 46.48,30.4 50.04,30.4 50.93,31.29 v50.93,35.73 | v58.42,89.07 v51.69,89.07
  Bottom 0.254: v60.71,89.07 v58.42,89.07 | v51.69,89.07 51.69,88.82 51.44,88.56 51.44,36.24 v50.93,35.73
ZX_ARD
  Top 0.254: R59.2 107.82,68.12 J2.8
ZX_ISO
  Top 0.254: U6.8 106.91,58.32 107.57,58.97 | 107.57,58.97 107.95,59.36 107.95,62.19 R59.1 | TP17.TP 110.49,56.05 107.57,58.97
(copper drawn outside any net)
  shapes: Top circle x3

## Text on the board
tPlace: PM1_ISO | RESET_ISO | GND_ISO | RESET | PM1 | GND_LIVE | ADE9000_RESET | IA | IB | SS_ADE | MISO_ADE | IC | MOSI_ADE | SCLK_ADE | IN | MOSI_ISO | GND | SCLK_ISO | SS_ISO | SCLK_ISO | MISO_ISO | MOSI_ISO | GND_ISO | MISO_ISO | ICSP | SS_ISO | ESP8266 Node MCU | PHASE A | 5V | 3V3_ISO | PHASE B | * | PHASE C | 5V | IRQ0_ISO | IRQ1_ISO | DREADY_ISO | ZX_ISO | GND_ISO | CAUTION! HIGH VOLTAGE | NEUTRAL | 3V3 | ADE9000 ARDUINO SHIELD | REV A.0 | DREADY | GND_LIVE | IRQ0 | IRQ1 | ZX
bPlace: MOSI_ISO | SCLK_ISO | MISO_ISO | SS_ISO
DrillLegend: DRILL LEGEND
FabDoc1: LAYER STACKUP: / --TOP SILKSCREEN / --TOP SOLDERMASK / --TOP LAYER / --BOTTOM LAYER / --BOTTOM SOLDERMASK / --BOTTOM SILKSCREEN / / NOMINAL FINISHED BOARD THICKNESS: 0.062" | PCB SPECIFICATIONS: / --SOLDERMASK: GREEN / --SILKSCREEN: WHITE / --MATERIAL: STANDARD FR4 / --SURFACE FINISH: ENIG / --FINISHED COPPER: 1 Oz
